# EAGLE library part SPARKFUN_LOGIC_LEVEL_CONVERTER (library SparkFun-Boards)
SparkFun Logic Level Converter -Bi-Directional This is the mechnical outline for the 3.3V - 5V bi directional logic level converter. *Note, the "LOCK" Package has the header pins staggered by an offset of 5 mils (off center line), so that when you slide a row of standard 0.1" headers into the PTH pads, it will hold position vertically. See the follwing turorial for more information on this type of special footprints: Sneaky Footprints SparkFun Products: SparkFun Logic Level Converter - Bi-Directional
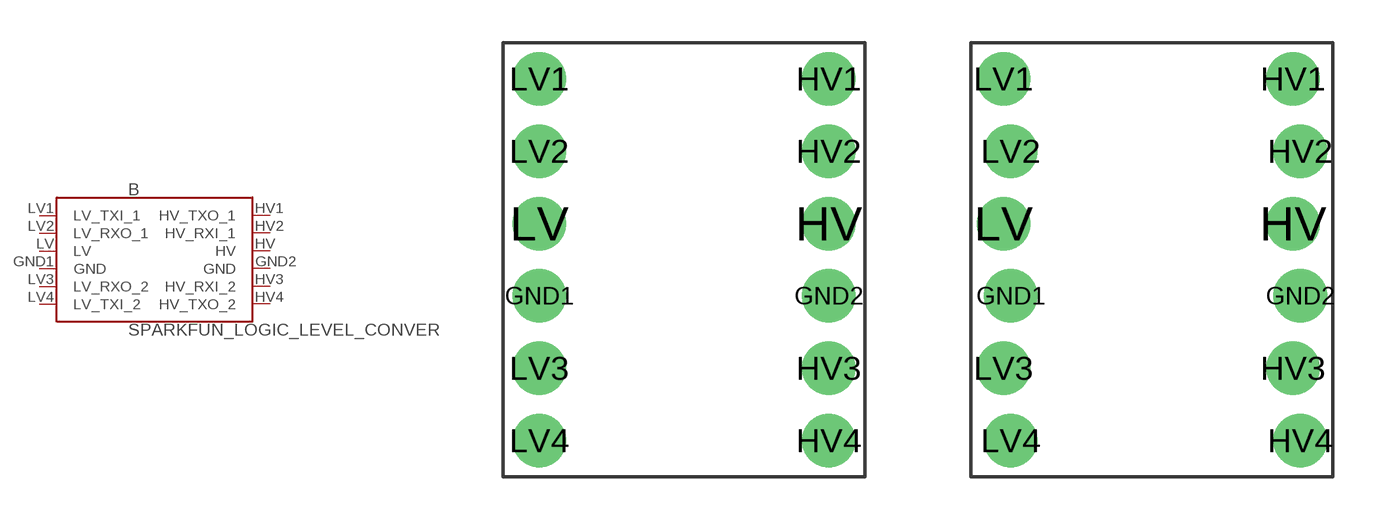
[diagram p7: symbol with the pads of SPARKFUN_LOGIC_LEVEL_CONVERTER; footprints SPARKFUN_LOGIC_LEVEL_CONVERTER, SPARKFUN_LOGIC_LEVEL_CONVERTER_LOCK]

Designator prefix B

## SPARKFUN_LOGIC_LEVEL_CONVERTER  [SPARKFUN_LOGIC_LEVEL_CONVERTER]
GND1  GND  pwr
GND2  GND  pwr
HV  HV  pwr
HV1  HV_TXO_1
HV2  HV_RXI_1
HV3  HV_RXI_2
HV4  HV_TXO_2
LV  LV  pwr
LV1  LV_TXI_1
LV2  LV_RXO_1
LV3  LV_RXO_2
LV4  LV_TXI_2

## SPARKFUN_LOGIC_LEVEL_CONVERTERLOCK  [SPARKFUN_LOGIC_LEVEL_CONVERTER_LOCK]
Pads as for SPARKFUN_LOGIC_LEVEL_CONVERTER

## Footprint SPARKFUN_LOGIC_LEVEL_CONVERTER (pad centres in mm)
SparkFun Logic Level Converter Specifications: Pin count:12 Pin pitch: 0.1" Area: 0.6x 0.5 " Example device(s): SparkFun Logic Level Converter
drill 1.016 pad 1.88: GND1 -5.08,-1.27; GND2 5.08,-1.27; HV 5.08,1.27; HV1 5.08,6.35; HV2 5.08,3.81; HV3 5.08,-3.81; HV4 5.08,-6.35; LV -5.08,1.27; LV1 -5.08,6.35; LV2 -5.08,3.81; LV3 -5.08,-3.81; LV4 -5.08,-6.35

## Footprint SPARKFUN_LOGIC_LEVEL_CONVERTER_LOCK (pad centres in mm)
drill 1.016 pad 1.88: GND1 -4.953,-1.27; GND2 5.207,-1.27; HV 4.953,1.27; HV1 4.953,6.35; HV2 5.207,3.81; HV3 4.953,-3.81; HV4 5.207,-6.35; LV -5.207,1.27; LV1 -5.207,6.35; LV2 -4.953,3.81; LV3 -5.207,-3.81; LV4 -4.953,-6.35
